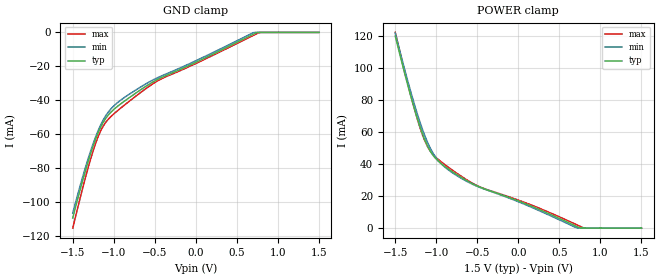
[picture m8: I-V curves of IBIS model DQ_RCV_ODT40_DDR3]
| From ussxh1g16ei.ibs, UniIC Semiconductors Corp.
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|   Model DQ_RCV_ODT40_DDR3
[Model] DQ_RCV_ODT40_DDR3
Model_type Input
Vinl =  0.615V
Vinh =  0.885V
C_comp   1.232pF   1.219pF   1.235pF
[Model Spec]
Vinh   0.885V   0.847V   0.922V
Vinl   0.615V   0.577V   0.652V
[Temperature Range]   25.000   95.000   -40.000
[Voltage Range]   1.500V   1.425V   1.575V
[GND_clamp]
|Voltage   I(typ)   I(min)   I(max)
-1.5V     -109.6mA   -106.7mA   -115.6mA
-1.314V   -76.53mA   -74.83mA   -80.19mA
-1.252V   -67.15mA   -65.75mA   -70.01mA
-1.19V    -59.17mA   -57.93mA   -61.48mA
-1.128V   -53.03mA   -51.65mA   -55.28mA
-1.066V   -48.73mA   -46.99mA   -51.25mA
-973mV    -44.39mA   -42.24mA   -47.03mA
-849mV    -39.87mA   -37.74mA   -42.13mA
-446mV    -27.29mA   -26.31mA   -28.09mA
701mV     -1.066mA   -167.7uA   -1.763mA
763mV     0A         0A         -281.8uA
1.5V      0A         0A         0A
[POWER_clamp]
|Voltage   I(typ)   I(min)   I(max)
-1.5V     119.8mA    121.5mA    122mA
-1.29V    78.46mA    81.2mA     78.71mA
-1.166V   58.41mA    61.19mA    57.81mA
-1.104V   50.89mA    53.17mA    50.58mA
-1.042V   45.55mA    46.9mA     46.01mA
-887mV    38.08mA    37.67mA    39.24mA
-701mV    31.8mA     31.22mA    32.52mA
-484mV    25.86mA    25.69mA    26.05mA
167mV     13.52mA    12.84mA    14.23mA
725mV     706uA      0A         1.785mA
818mV     0A         0A         0A
1.5V      0A         0A         0A
